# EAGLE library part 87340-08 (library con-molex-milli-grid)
RECEPTACAL
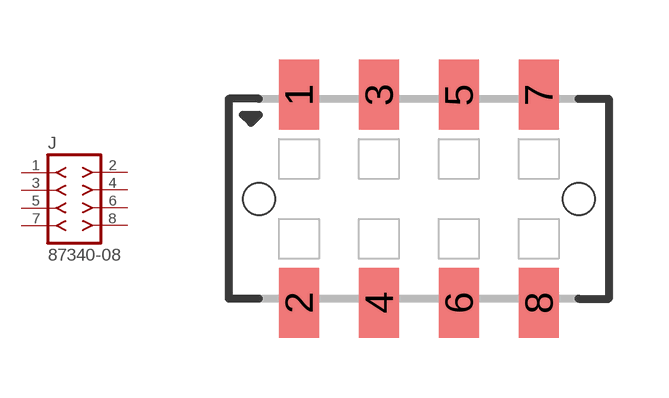
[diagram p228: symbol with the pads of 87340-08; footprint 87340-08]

Designator prefix J

## 87340-08  [87340-08]
1  1  pas
2  2  pas
3  3  pas
4  4  pas
5  5  pas
6  6  pas
7  7  pas
8  8  pas

## Footprint 87340-08 (pad centres in mm)
RECEPTACAL SMD Dual Row, Vertical, Low Profile
smd 1 x 1.75: 1 -3,2.6; 2 -3,-2.6; 3 -1,2.6; 4 -1,-2.6; 5 1,2.6; 6 1,-2.6; 7 3,2.6; 8 3,-2.6
hole 0.8 at -4,0
hole 0.8 at 4,0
